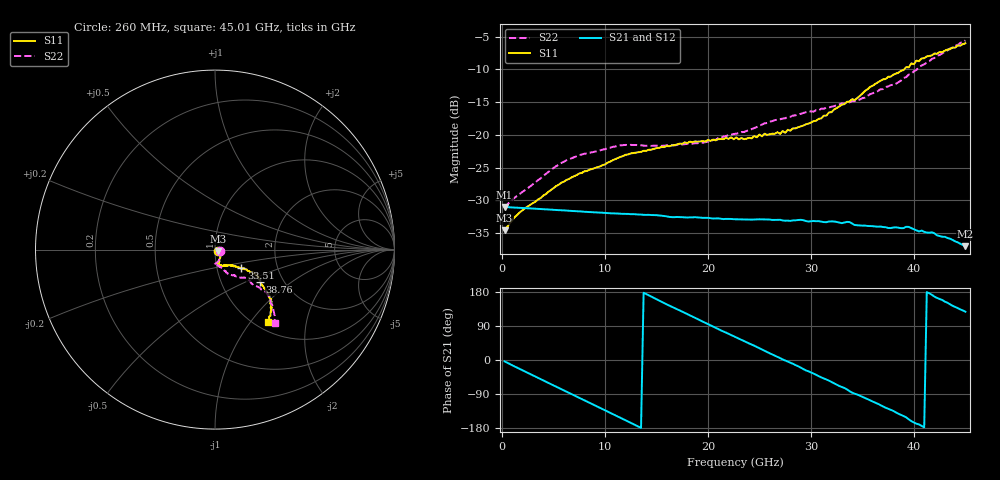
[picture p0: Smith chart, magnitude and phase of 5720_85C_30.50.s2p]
! Device:  ADRF5720
! Description: 0.5dB LSB GaAs MMIC 6-bit Digital Attenuator
! Frequency:  0.000009 -  40 GHz
! Ports:
!	RF1	= Port 1
!	RF2	= Port 2
! Vdd:  3.3 Volt
! Vss:  -3.3 Volt
! Control:  0/3.3 Volt
! State:  30.50 dB attenuation
! Data:  The device was measured using G-S-G Probes on a matrix board.
!  Data was collected using an calibrated 4 port network analyzer.
!  The reference plane for this measurement is at the launchers.
! Note:  Analog Devices supplies this data as a sample of measured data
!  for this product.  Your particular data for this product may vary.
!  Data was taken at 85 degrees C.
!  Analog Devices reserves the right to change this data at anytime.
# GHZ S DB R 45.0
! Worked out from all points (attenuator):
!   180 points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, 260 MHz to 45.01 GHz, reference 45 ohm
!   highest |S21| = -31.03 dB at 260 MHz (marker M1); lowest = -37.0 dB at 45.01 GHz (marker M2)
!   lowest |S11| = -34.6 dB at 260 MHz (marker M3), VSWR 1.04, Z = 46.6 - j0.718 ohm
!   |S11| at or under -10 dB: start of sweep to 39.07 GHz
!   |S22| runs from -31.2 to -5.6 dB; largest |S21 - S12| = 0.00027
!   S11 on the Smith chart (normalised r, x): 260 MHz: 1.03, -0.02; 33.51 GHz: 1.31, -0.28; 38.76 GHz: 1.53, -0.61; 45.01 GHz: 1.13, -1.22
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0.26  -34.57 -24.4  -31.03 -3.7  -31.03 -3.7  -31.20 -17.9
2.26  -31.20 -9.5  -31.21 -30.8  -31.19 -30.7  -28.41 -25.7
5.26  -27.84 -42.5  -31.49 -70.3  -31.47 -70.3  -24.80 -64.0
7.76  -25.82 -54.8  -31.72 -103.2  -31.71 -103.1  -23.00 -78.2
11.51  -23.37 -69.3  -32.06 -152.5  -32.05 -152.4  -21.61 -91.5
15.26  -21.99 -76.0  -32.33 156.9  -32.32 157.1  -21.67 -92.5
19.51  -20.95 -77.3  -32.69 101.2  -32.67 101.4  -21.20 -81.8
22.76  -20.39 -72.2  -32.91 59.3  -32.89 59.5  -19.81 -72.6
23.51  -20.66 -71.7  -32.94 49.8  -32.93 50.0  -19.57 -70.4
25.51  -19.82 -64.4  -32.92 24.4  -32.90 24.6  -18.24 -68.2
27.01  -19.85 -59.1  -32.98 4.9  -32.97 5.2  -17.62 -64.2
30.26  -17.91 -45.2  -33.17 -35.8  -33.15 -35.6  -16.45 -61.7
33.51  -14.94 -35.3  -33.31 -77.6  -33.29 -77.4  -15.09 -54.5
34.26  -14.67 -36.3  -33.79 -88.9  -33.78 -88.6  -14.84 -52.3
35.76  -12.67 -32.3  -33.95 -106.3  -33.92 -105.9  -13.78 -49.2
37.76  -11.10 -32.0  -34.25 -131.6  -34.23 -131.3  -12.39 -42.6
38.76  -10.20 -35.5  -34.27 -144.9  -34.23 -144.1  -11.71 -42.0
39.51  -9.68 -36.8  -34.08 -156.6  -34.06 -156.3  -10.78 -42.7
39.76  -9.07 -38.0  -34.26 -161.3  -34.26 -161.2  -10.67 -42.9
42.01  -7.55 -41.6  -35.05 167.1  -35.05 167.7  -8.24 -40.7
43.51  -6.91 -45.4  -35.87 147.3  -35.82 147.5  -6.80 -45.2
45.01  -6.01 -54.2  -37.02 127.4  -37.00 127.1  -5.57 -50.6
